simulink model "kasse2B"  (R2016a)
settings: Solver=ode45  StartTime=0.0  StopTime=100  FixedStep=0.001  MaxStep=2  RelTol=1e-3
undefined symbols (not defined in the file or in its folder): tAb, z0
libraries: simulink x2

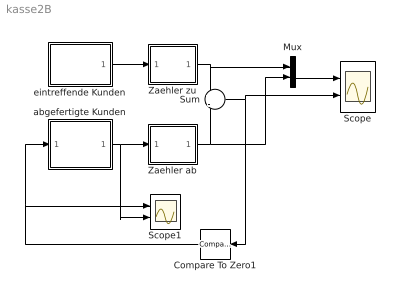
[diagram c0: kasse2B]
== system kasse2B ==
  Compare To Zero1 : simulink/Logic and Bit Operations/Compare To Zero  relop=<=  OutDataTypeStr=uint8
  Mux : Mux  Inputs=2
  Scope : Scope  NumInputPorts=2
  Scope1 : Scope  NumInputPorts=2
  Sum : Sum  Inputs=+|-
  Zaehler ab : Subsystem
  Zaehler zu : Subsystem
  abgefertigte Kunden : Subsystem
  eintreffende Kunden : Subsystem
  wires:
  Zaehler zu/1(Out) -> Sum/1, Mux/1
  eintreffende Kunden/1(Out1) -> Zaehler zu/1(In)
  abgefertigte Kunden/1(Out) -> Scope1/2, Zaehler ab/1(In)
  Zaehler ab/1(Out) -> Sum/2, Mux/2
  Sum/1 -> Compare To Zero1/1, Scope/2
  Compare To Zero1/1 -> abgefertigte Kunden/1(In1), Scope1/1
  Mux/1 -> Scope/1

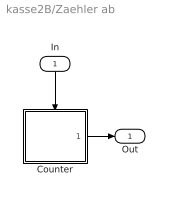
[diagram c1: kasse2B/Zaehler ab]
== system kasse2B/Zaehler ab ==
  In : Inport
  Counter : Subsystem
  Out : Outport
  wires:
  In/1 -> Counter/Trigger
  Counter/1(Out) -> Out/1

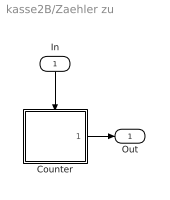
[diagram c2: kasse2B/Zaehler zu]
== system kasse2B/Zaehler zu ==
  In : Inport
  Counter : Subsystem
  Out : Outport
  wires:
  In/1 -> Counter/Trigger
  Counter/1(Out) -> Out/1

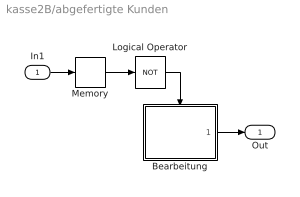
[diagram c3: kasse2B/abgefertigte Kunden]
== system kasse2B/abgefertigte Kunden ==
  In1 : Inport
  Bearbeitung : Subsystem
  Logical Operator : Logic  Operator=NOT  AllPortsSameDT=off  OutDataTypeStr=boolean
  Memory : Memory
  Out : Outport
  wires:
  Logical Operator/1 -> Bearbeitung/Enable
  Memory/1 -> Logical Operator/1
  In1/1 -> Memory/1
  Bearbeitung/1(Out1) -> Out/1

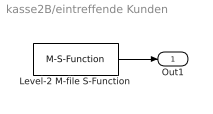
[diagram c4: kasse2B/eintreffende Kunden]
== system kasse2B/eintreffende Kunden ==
  Level-2 M-file S-Function : M-S-Function  FunctionName=sfun_poisson  Parameters=lambda
  Out1 : Outport
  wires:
  Level-2 M-file S-Function/1 -> Out1/1

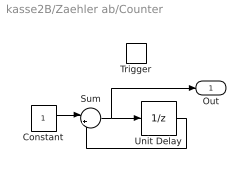
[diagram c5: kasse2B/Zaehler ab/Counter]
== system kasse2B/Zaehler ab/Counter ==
  Trigger : TriggerPort  TriggerType=falling  VariantControl=Variant
  Constant : Constant
  Sum : Sum  Inputs=|++
  Unit Delay : UnitDelay  InitialCondition=z0  SampleTime=-1
  Out : Outport  InitialOutput=z0
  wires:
  Unit Delay/1 -> Sum/2
  Sum/1 -> Out/1, Unit Delay/1
  Constant/1 -> Sum/1

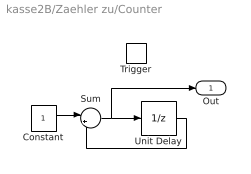
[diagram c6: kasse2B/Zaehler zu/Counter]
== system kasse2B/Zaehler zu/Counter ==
  Trigger : TriggerPort  TriggerType=falling  VariantControl=Variant
  Constant : Constant
  Sum : Sum  Inputs=|++
  Unit Delay : UnitDelay  InitialCondition=z0  SampleTime=-1
  Out : Outport  InitialOutput=z0
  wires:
  Unit Delay/1 -> Sum/2
  Sum/1 -> Out/1, Unit Delay/1
  Constant/1 -> Sum/1

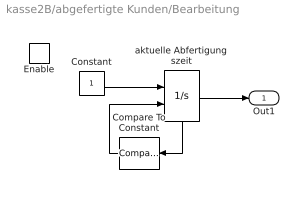
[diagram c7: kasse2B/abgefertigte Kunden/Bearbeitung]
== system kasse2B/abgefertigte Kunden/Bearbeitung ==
  Enable : EnablePort  StatesWhenEnabling=reset
  Compare To Constant : simulink/Logic and Bit Operations/Compare To Constant  SystemSampleTime=-1  relop=>=  const=tAb  LogicOutDataTypeMode=boolean
  Constant : Constant
  aktuelle Abfertigungszeit : Integrator  ExternalReset=rising  ShowStatePort=on
  Out1 : Outport  OutputWhenDisabled=reset  InitialOutput=0
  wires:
  Compare To Constant/1 -> aktuelle Abfertigungszeit/2
  aktuelle Abfertigungszeit/1 -> Out1/1
  Constant/1 -> aktuelle Abfertigungszeit/1
  aktuelle Abfertigungszeit/State -> Compare To Constant/1
